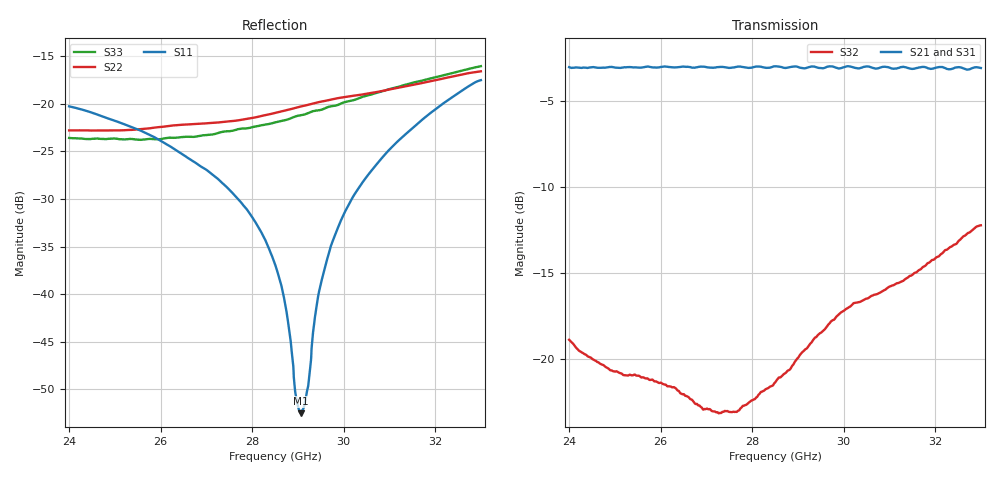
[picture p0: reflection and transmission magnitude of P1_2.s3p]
!The following data was pulled from an Agilent PNA
!This sNp file was generated from the data in the RF Test software
!NOTE:  Smoothing/Math/Corrections applied on any given trace ARE included in the data saved here
# MHz S dB R 50
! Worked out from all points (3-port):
!   1601 points, 24 GHz to 33 GHz, reference 50 ohm
!   strongest paths, dB at 24 GHz, 26.25 GHz, 28.5 GHz, 30.75 GHz, 33 GHz:
!     S21: -3.0, -3.0, -3.0, -3.1, -3.1
!     S31: -3.0, -3.0, -3.2, -3.2, -3.3
!     S32: -18.9, -21.6, -21.4, -16.2, -12.2
!   lowest |S11| = -52.5 dB at 29.06 GHz (marker M1), VSWR 1.00, Z = 50.2 + j0.091 ohm
!   |S11| at or under -10 dB: start of sweep to end of sweep
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24000  -20.26 23.5  -3.14 153.7  -3.13 152.7
       -3.01 153.6  -22.79 -172.7  -18.83 82.6
       -3.01 152.1  -18.88 82.2  -23.58 -176.5
27031.88  -27.04 -5.1  -3.02 124.0  -3.06 122.2
          -3.02 123.5  -22.03 157.6  -22.90 5.1
          -3.06 121.9  -22.91 4.8  -23.26 146.3
28500  -36.85 -18.0  -3.04 108.9  -3.16 106.9
       -2.96 108.8  -20.95 146.2  -21.34 -35.2
       -3.17 106.7  -21.37 -35.2  -21.96 132.6
28725  -41.09 -21.0  -3.06 106.4  -3.17 104.5
       -3.05 106.5  -20.70 144.2  -20.79 -41.8
       -3.11 104.5  -20.82 -41.9  -21.70 130.8
29062.5  -52.51 22.5  -3.04 102.8  -3.17 101.0
         -3.05 102.7  -20.28 141.0  -19.69 -50.9
         -3.14 101.2  -19.70 -51.1  -21.20 127.7
29208.75  -50.00 102.4  -3.07 101.4  -3.20 99.6
          -3.04 101.9  -20.11 139.5  -19.32 -55.2
          -3.14 99.2  -19.33 -55.4  -21.00 126.0
29495.62  -39.03 162.1  -3.05 98.4  -3.20 96.5
          -3.06 98.4  -19.77 136.5  -18.46 -64.2
          -3.14 96.5  -18.48 -64.5  -20.64 123.4
30125.62  -30.45 154.0  -3.04 91.8  -3.22 90.0
          -2.96 91.8  -19.20 129.2  -16.94 -82.4
          -3.27 90.0  -16.97 -82.7  -19.71 116.5
31183.12  -23.93 142.9  -3.05 80.2  -3.25 78.6
          -3.06 80.9  -18.33 119.2  -15.56 -105.0
          -3.25 78.5  -15.58 -105.2  -18.23 105.2
33000  -17.50 126.3  -3.17 60.2  -3.36 58.8
       -3.06 60.5  -16.58 102.9  -12.14 -135.1
       -3.32 59.3  -12.21 -135.2  -16.04 86.7
